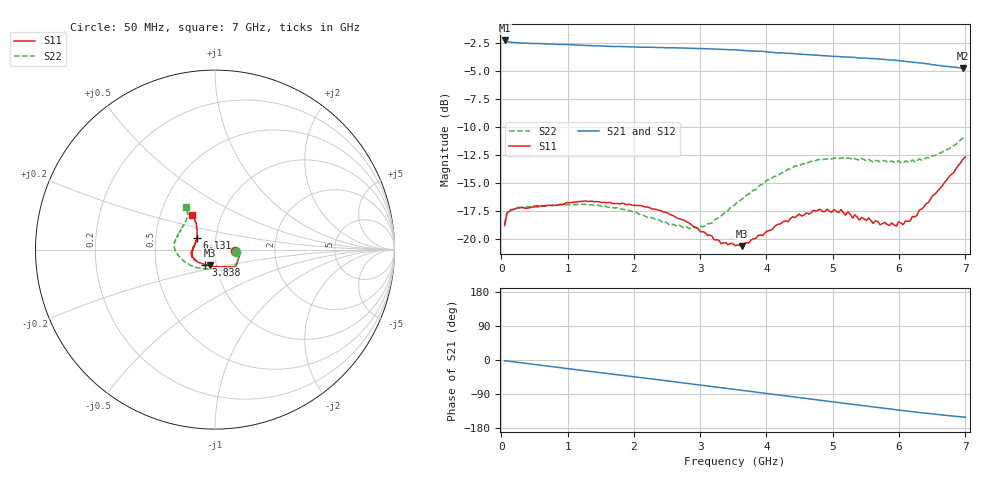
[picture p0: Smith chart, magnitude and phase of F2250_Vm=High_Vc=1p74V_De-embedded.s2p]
! Integrated Device Technology
! Corporate Headquarters
! 6024 Silver Creek Valley Road
! San Jose, CA 95138  USA
! Phone:  1-408-284-8200
! Toll Free:  1-800-223-1366
! Webpage:  http://www.idt.com/
! Timing and RF Division
! 515 Groton Road, Suite 102
! Westford, MA 01886-6024
! Device:  F2250
! Description: Voltage Variable RF Attenuator
! Frequency:  50.0 -  6000.00 MHz
! Package:  3x3 mm Thin QFN Plastic Package: 16 pin
! Ports:  2 RF, 3 DC
!  Pin  1  = GND
!  Pin  2  = NC
!  Pin  3  = RF1  = Port 1
!  Pin  4  = NC
!  Pin  5  = GND
!  Pin  6  = GND
!  Pin  7  = GND
!  Pin  8  = GND
!  Pin  9  = NC
!  Pin 10  = RF2  = Port 2
!  Pin 11  = NC
!  Pin 12  = GND
!  Pin 13  = GND
!  Pin 14  = VCNTRL
!  Pin 15  = VDD
!  Pin 16  = VMODE
! Vcntrl:  1.740 Volts
! Vmode:  +3.300 Volts
! Vdd:  +3.30  Volts
! Current:  1.325 mA
! Data:  The device was measured on a the F2250 evaluation board which has
!  individual transmission lines to the RF pins.  Data was collected
!  using a calibrated network analyzer.  The evaluation board was
!  de-embedded using a TRL calibration technique.
!  The reference plane is the edge of the package pin.
! Misc:  SN 10
!  Action Tracker AT0258
! Date Measured:  2014-11-26
! Date:  2015-10-15  MJV
! Note:
!  Integrated Device Technology supplies this data as a sample of measured
!  data at the package pin for this product.  Your particular data for this
!  product may vary.
!  Data was taken at 25 degrees C.
!  Integrated Device Technology reserves the right to change this data at anytime.
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# GHz S dB R 50
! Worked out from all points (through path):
!   201 points, 50 MHz to 7 GHz, reference 50 ohm
!   highest |S21| = -2.30 dB at 50 MHz (marker M1); lowest = -4.8 dB at 6.965 GHz (marker M2)
!   group delay of S21, straight-line fit = 60.6 ps
!   lowest |S11| = -20.7 dB at 3.629 GHz (marker M3), VSWR 1.20, Z = 46.7 - j8.33 ohm
!   |S11| at or under -10 dB: start of sweep to end of sweep
!   |S22| runs from -19.1 to -10.9 dB; largest |S21 - S12| = 0.0028
!   S11 on the Smith chart (normalised r, x): 50 MHz: 1.26, -0.02; 3.838 GHz: 0.89, -0.15; 6.131 GHz: 0.81, +0.11; 7 GHz: 0.72, +0.30
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0.05  -18.84 -4.6  -2.30 -1.9  -2.31 -1.9  -18.74 -5.8
0.08475  -17.76 -4.2  -2.41 -2.6  -2.41 -2.6  -17.65 -5.4
0.2585  -17.21 -9.7  -2.50 -6.4  -2.51 -6.4  -17.29 -12.5
1.2315  -16.66 -35.7  -2.74 -27.8  -2.76 -27.8  -16.92 -47.8
2.37825  -17.47 -45.7  -2.94 -52.3  -2.94 -52.3  -18.31 -72.8
2.969  -19.12 -59.7  -3.01 -65.4  -3.01 -65.4  -19.06 -100.4
3.3165  -20.46 -81.9  -3.09 -73.3  -3.10 -73.3  -17.97 -123.4
3.525  -20.64 -98.0  -3.14 -78.0  -3.14 -78.0  -16.97 -135.2
3.62925  -20.67 -106.9  -3.18 -80.3  -3.19 -80.4  -16.49 -140.4
3.83775  -19.98 -122.0  -3.25 -85.0  -3.26 -85.0  -15.62 -150.2
4.32425  -18.49 -147.6  -3.45 -95.7  -3.45 -95.8  -13.80 -169.0
4.7065  -17.46 -161.6  -3.59 -104.2  -3.59 -104.2  -13.11 -179.0
5.1235  -17.40 -172.3  -3.75 -113.2  -3.75 -113.3  -12.80 170.9
5.29725  -18.17 -177.4  -3.81 -116.9  -3.81 -117.0  -12.94 167.3
5.332  -17.87 -179.1  -3.82 -117.8  -3.82 -117.8  -12.85 166.4
5.4015  -18.35 179.8  -3.87 -119.2  -3.85 -119.3  -13.01 164.4
5.5405  -18.15 173.7  -3.92 -122.2  -3.90 -122.3  -12.92 160.7
5.85325  -18.83 161.8  -4.05 -128.9  -4.04 -129.0  -13.17 152.4
6.13125  -18.47 147.5  -4.20 -134.8  -4.20 -134.9  -13.17 144.7
6.54825  -15.99 130.6  -4.49 -143.4  -4.50 -143.5  -12.57 131.3
6.96525  -12.89 123.6  -4.79 -150.4  -4.81 -150.5  -11.01 125.7
7  -12.71 123.2  -4.77 -150.9  -4.80 -151.0  -10.87 124.8
